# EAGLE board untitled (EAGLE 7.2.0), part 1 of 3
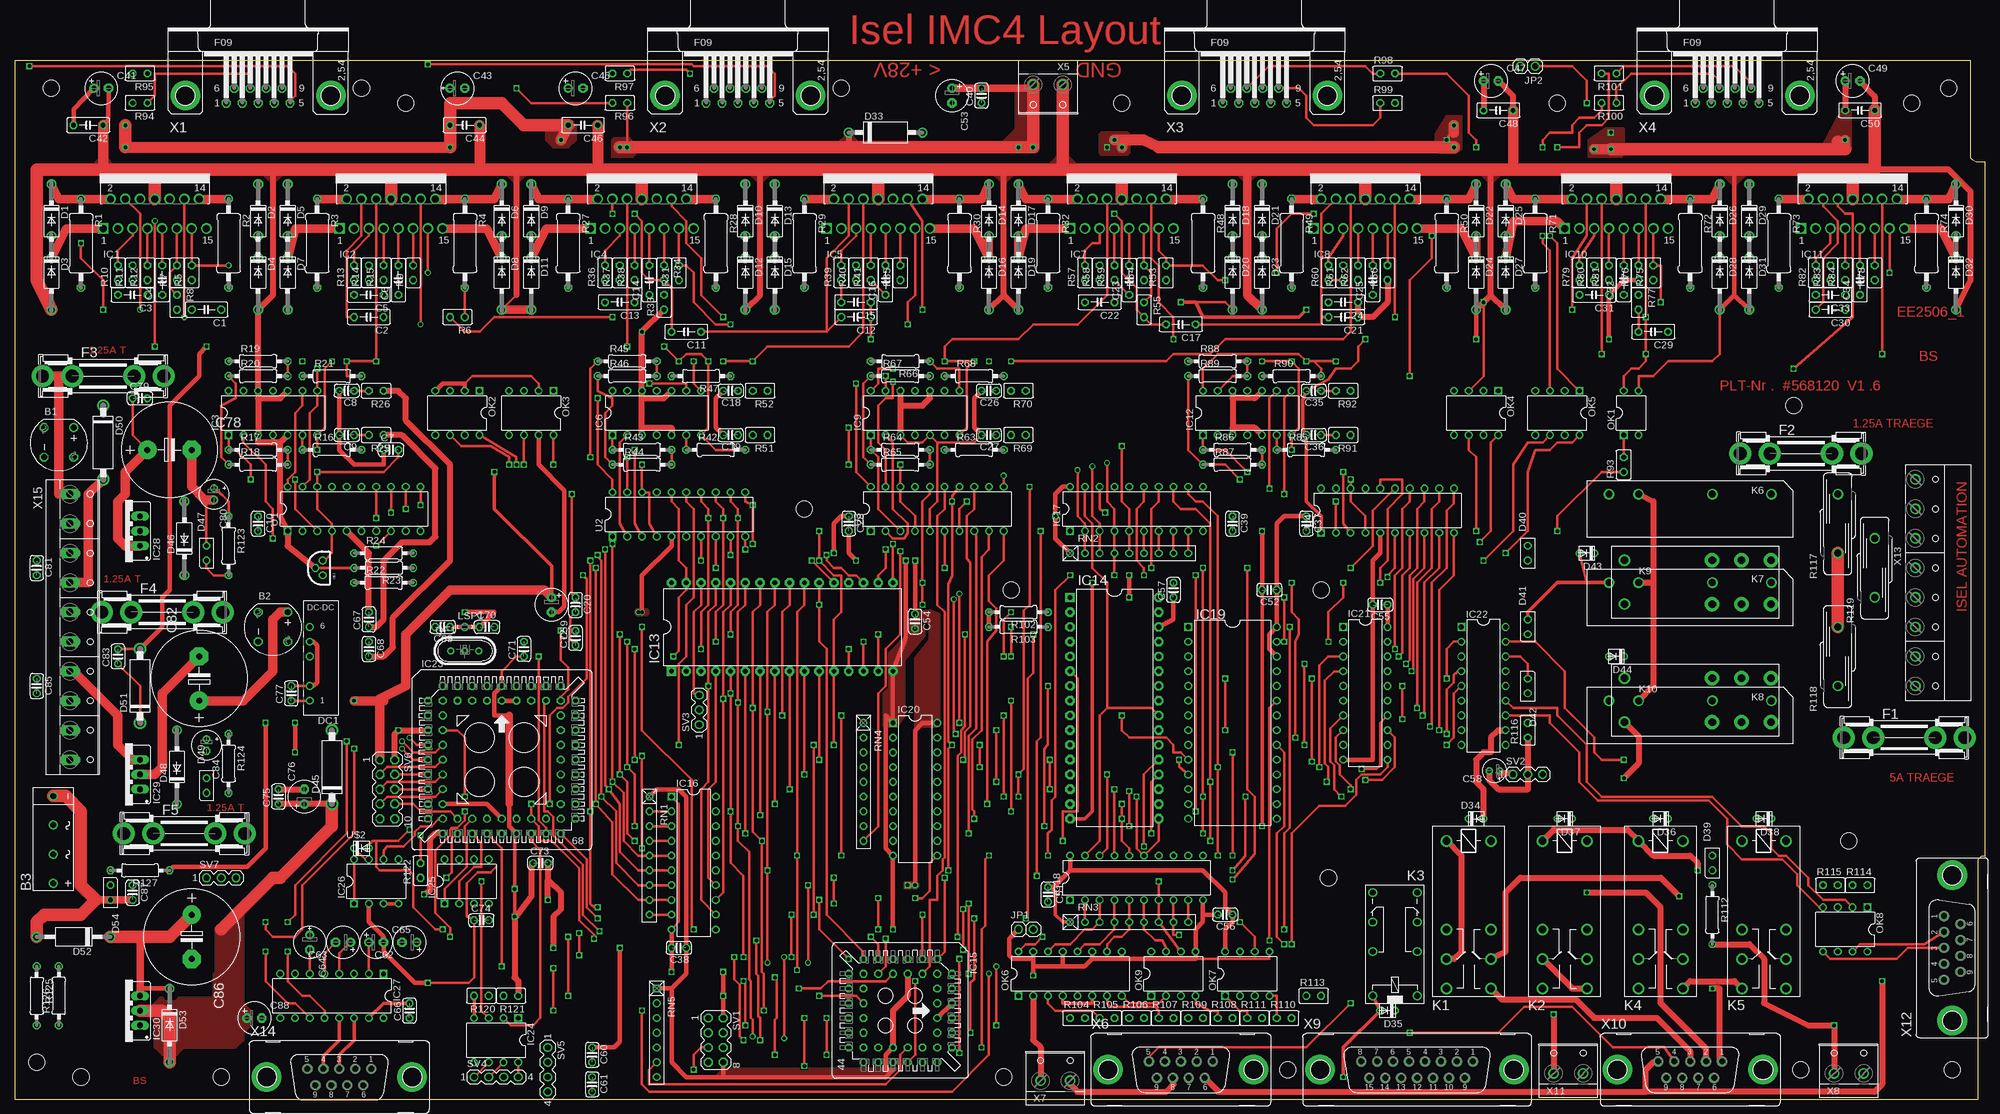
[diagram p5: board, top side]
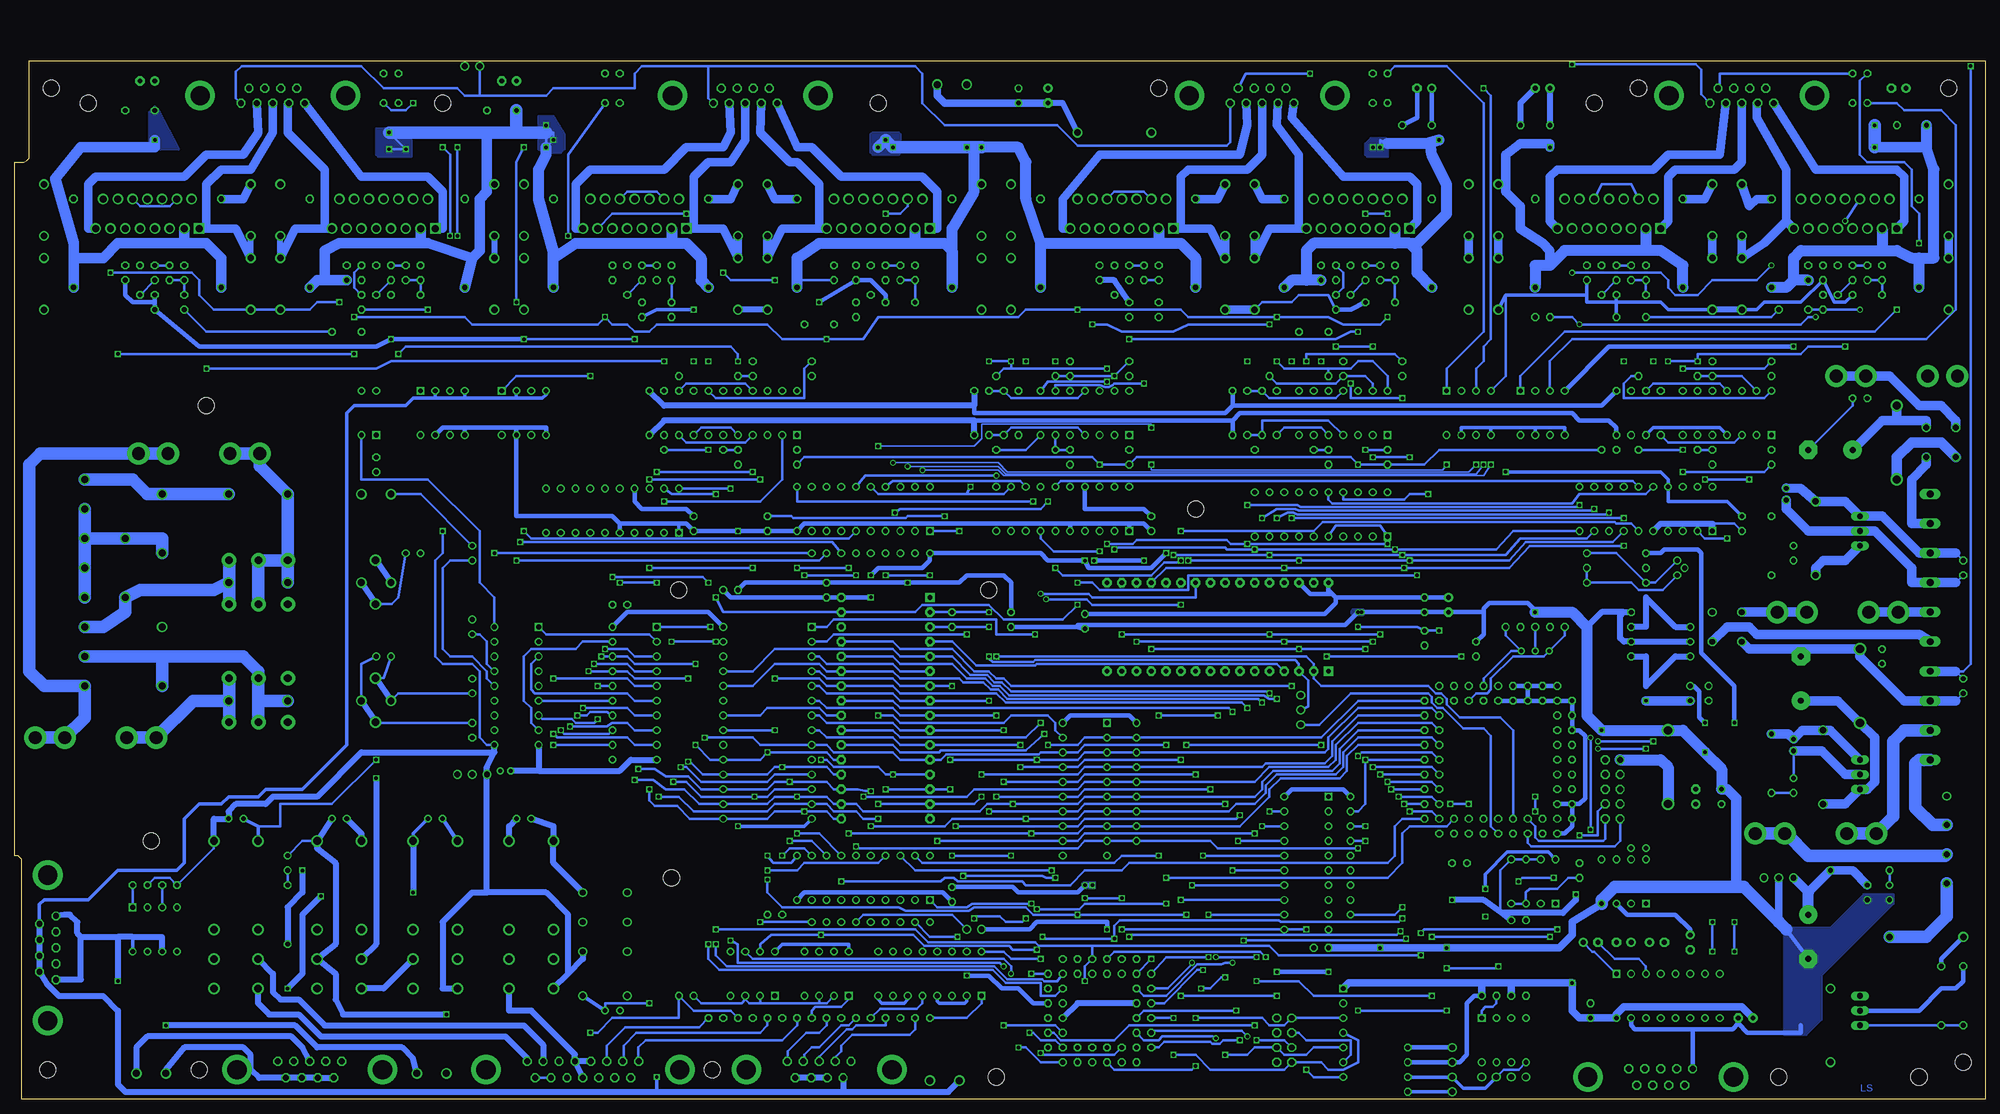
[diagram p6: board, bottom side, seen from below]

Size 339.09 x 178.74 mm. Coordinates in mm from the lower left corner, seen from the top.
Outline: 0,0 337.82,0 337.82,41.28 338.46,41.91 339.09,41.91 339.09,161.29 337.5,161.29 336.87,161.61 336.55,161.93 336.53,162.26 336.53,178.74 0,178.74 0,0
Copper layers (1*16): Top 0.035mm / dielectric 1.5mm / Bottom 0.035mm
Design rules "default": minimum track width 10mil, minimum drill 24mil, track to track 8mil, track to pad 8mil, pad to pad 8mil, via to via 8mil, smd to smd 8mil, copper to edge 40mil, drill to drill 8mil, minimum pad ring 10mil, minimum via ring 8mil, stop-mask expansion 4mil, vias tented up to drill 0mil, thermal gap 10mil
Holes 2.8 mm at 171.45,87.63 224.79,87.63 219.07,5.08 170.18,3.81 307.34,5.08 333.38,5.08 226.06,38.1 35.56,3.81 306.07,119.38 315.6,44.45 326.39,171.45 332.74,173.99 265.43,171.45 142.24,173.99 190.5,171.45 59.69,173.99 67.31,171.45 6.35,173.99 135.89,101.6 3.81,6.35 11.43,3.81

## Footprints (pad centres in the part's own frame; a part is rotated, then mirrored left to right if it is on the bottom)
RB1A = drill 1.016: + -2.54,2.54 | drill 1.016 octagon: - 2.54,-2.54; AC1 2.54,2.54; AC2 -2.54,-2.54
2KBB-R = drill 1.016: + -7.62,0; - 7.391,0; AC1 -2.616,0; AC2 2.413,0
C050-025X075 = drill 0.813 octagon: 1 -2.54,0; 2 2.54,0
C025-024X044 = drill 0.813 octagon: 1 -1.27,0; 2 1.27,0
E2,5-6 = drill 0.813 pad 1.6: + -1.27,0 | drill 0.813 pad 1.6 octagon: - 1.27,0
E2,5-6E = drill 0.813 pad 1.575: + -1.27,0 | drill 0.813 pad 1.575 octagon: - 1.27,0
E1,8-4 = drill 0.711 pad 1.168: + -0.889,0 | drill 0.711 pad 1.168 octagon: - 0.889,0
E7,5-16 = drill 1.016 pad 3.15: + -3.81,0 | drill 1.016 pad 3.15 octagon: - 3.81,0
E2-5 = drill 0.813 pad 1.27: + -1.016,0 | drill 0.813 pad 1.27 octagon: - 1.016,0
DO41-10 = drill 1.118: A 6.35,0; C -6.35,0
DO15-12 = drill 1.118: A 6.35,0; C -6.35,0
DO41-10' = drill 0.8: A 1.27,0; C -1.27,0
U57X32 = drill 0.813: A 1.27,0; K -1.27,0
C1702-15 = drill 1.397: A 5.08,0; C -7.62,0
P1-12E = drill 1.118: A 6.35,0; C -6.35,0
NMA = drill 0.813: 1 0,6.35; 2 0,3.81; 4 0,-1.27; 5 0,-3.81; 6 0,-6.35
SHK20L = drill 2.2 pad 3.81: 1A -10.414,0; 1B -5.334,0; 2A 10.414,0; 2B 5.334,0
MULTIWATT-15 = drill 1.2 square: 1 -8.89,-7.62 | drill 1.2: 2 -7.62,-2.54; 3 -6.35,-7.62; 4 -5.08,-2.54; 5 -3.81,-7.62; 6 -2.54,-2.54; 7 -1.27,-7.62; 8 0,-2.54; 9 1.27,-7.62; 10 2.54,-2.54; 11 3.81,-7.62; 12 5.08,-2.54; 13 6.35,-7.62; 14 7.62,-2.54; 15 8.89,-7.62
DIL14 = drill 0.813 square: 1 -7.62,-3.81 | drill 0.813: 2 -5.08,-3.81; 3 -2.54,-3.81; 4 0,-3.81; 5 2.54,-3.81; 6 5.08,-3.81; 7 7.62,-3.81; 8 7.62,3.81; 9 5.08,3.81; 10 2.54,3.81; 11 0,3.81; 12 -2.54,3.81; 13 -5.08,3.81; 14 -7.62,3.81
DIL32-3 = drill 0.813 pad 1.6 square: 1 -16.51,-7.62 | drill 0.813 pad 1.6 octagon: 2 -13.97,-7.62; 3 -11.43,-7.62; 4 -8.89,-7.62; 5 -6.35,-7.62; 6 -3.81,-7.62; 7 -1.27,-7.62; 8 1.27,-7.62; 9 3.81,-7.62; 10 6.35,-7.62; 11 8.89,-7.62; 12 11.43,-7.62; 13 13.97,-7.62; 14 16.51,-7.62; 15 19.05,-7.62; 16 21.59,-7.62; 17 21.59,7.62; 18 19.05,7.62; 19 16.51,7.62; 20 13.97,7.62; 21 11.43,7.62; 22 8.89,7.62; 23 6.35,7.62; 24 3.81,7.62; 25 1.27,7.62; 26 -1.27,7.62; 27 -3.81,7.62; 28 -6.35,7.62; 29 -8.89,7.62; 30 -11.43,7.62; 31 -13.97,7.62; 32 -16.51,7.62
S44 = drill 0.813: 1 1.27,6.35 | drill 0.813 octagon: 2 -1.27,8.89; 3 -1.27,6.35; 4 -3.81,8.89; 5 -3.81,6.35; 6 -6.35,8.89; 7 -8.89,6.35; 8 -6.35,6.35; 9 -8.89,3.81; 10 -6.35,3.81; 11 -8.89,1.27; 12 -6.35,1.27; 13 -8.89,-1.27; 14 -6.35,-1.27; 15 -8.89,-3.81; 16 -6.35,-3.81; 17 -8.89,-6.35; 18 -6.35,-8.89; 19 -6.35,-6.35; 20 -3.81,-8.89; 21 -3.81,-6.35; 22 -1.27,-8.89; 23 -1.27,-6.35; 24 1.27,-8.89; 25 1.27,-6.35; 26 3.81,-8.89; 27 3.81,-6.35; 28 6.35,-8.89; 29 8.89,-6.35; 30 6.35,-6.35; 31 8.89,-3.81; 32 6.35,-3.81; 33 8.89,-1.27; 34 6.35,-1.27; 35 8.89,1.27; 36 6.35,1.27; 37 8.89,3.81; 38 6.35,3.81; 39 8.89,6.35; 40 6.35,8.89; 41 6.35,6.35; 42 3.81,8.89; 43 3.81,6.35; 44 1.27,8.89
DIL20 = drill 0.813 square: 1 -11.43,-3.81 | drill 0.813: 2 -8.89,-3.81; 3 -6.35,-3.81; 4 -3.81,-3.81; 5 -1.27,-3.81; 6 1.27,-3.81; 7 3.81,-3.81; 8 6.35,-3.81; 9 8.89,-3.81; 10 11.43,-3.81; 11 11.43,3.81; 12 8.89,3.81; 13 6.35,3.81; 14 3.81,3.81; 15 1.27,3.81; 16 -1.27,3.81; 17 -3.81,3.81; 18 -6.35,3.81; 19 -8.89,3.81; 20 -11.43,3.81
DIL28-6 = drill 0.813 square: 1 -16.51,-7.62 | drill 0.813: 2 -13.97,-7.62; 3 -11.43,-7.62; 4 -8.89,-7.62; 5 -6.35,-7.62; 6 -3.81,-7.62; 7 -1.27,-7.62; 8 1.27,-7.62; 9 3.81,-7.62; 10 6.35,-7.62; 11 8.89,-7.62; 12 11.43,-7.62; 13 13.97,-7.62; 14 16.51,-7.62; 15 16.51,7.62; 16 13.97,7.62; 17 11.43,7.62; 18 8.89,7.62; 19 6.35,7.62; 20 3.81,7.62; 21 1.27,7.62; 22 -1.27,7.62; 23 -3.81,7.62; 24 -6.35,7.62; 25 -8.89,7.62; 26 -11.43,7.62; 27 -13.97,7.62; 28 -16.51,7.62
DIL18 = drill 0.813 square: 1 -10.16,-3.81 | drill 0.813: 2 -7.62,-3.81; 3 -5.08,-3.81; 4 -2.54,-3.81; 5 0,-3.81; 6 2.54,-3.81; 7 5.08,-3.81; 8 7.62,-3.81; 9 10.16,-3.81; 10 10.16,3.81; 11 7.62,3.81; 12 5.08,3.81; 13 2.54,3.81; 14 0,3.81; 15 -2.54,3.81; 16 -5.08,3.81; 17 -7.62,3.81; 18 -10.16,3.81
S68 = drill 0.813: 1 0,12.7 | drill 0.813 octagon: 2 0,10.16; 3 -2.54,12.7; 4 -2.54,10.16; 5 -5.08,12.7; 6 -5.08,10.16; 7 -7.62,12.7; 8 -7.62,10.16; 9 -10.16,12.7; 10 -12.7,10.16; 11 -10.16,10.16; 12 -12.7,7.62; 13 -10.16,7.62; 14 -12.7,5.08; 15 -10.16,5.08; 16 -12.7,2.54; 17 -10.16,2.54; 18 -12.7,0; 19 -10.16,0; 20 -12.7,-2.54; 21 -10.16,-2.54; 22 -12.7,-5.08; 23 -10.16,-5.08; 24 -12.7,-7.62; 25 -10.16,-7.62; 26 -12.7,-10.16; 27 -10.16,-12.7; 28 -10.16,-10.16; 29 -7.62,-12.7; 30 -7.62,-10.16; 31 -5.08,-12.7; 32 -5.08,-10.16; 33 -2.54,-12.7; 34 -2.54,-10.16; 35 0,-12.7; 36 0,-10.16; 37 2.54,-12.7; 38 2.54,-10.16; 39 5.08,-12.7; 40 5.08,-10.16; 41 7.62,-12.7; 42 7.62,-10.16; 43 10.16,-12.7; 44 12.7,-10.16; 45 10.16,-10.16; 46 12.7,-7.62; 47 10.16,-7.62; 48 12.7,-5.08; 49 10.16,-5.08; 50 12.7,-2.54; 51 10.16,-2.54; 52 12.7,0; 53 10.16,0; 54 12.7,2.54; 55 10.16,2.54; 56 12.7,5.08; 57 10.16,5.08; 58 12.7,7.62; 59 10.16,7.62; 60 12.7,10.16; 61 10.16,12.7; 62 10.16,10.16; 63 7.62,12.7; 64 7.62,10.16; 65 5.08,12.7; 66 5.08,10.16; 67 2.54,12.7; 68 2.54,10.16
DIL08 = drill 0.813 square: 1 -3.81,-3.81 | drill 0.813: 2 -1.27,-3.81; 3 1.27,-3.81; 4 3.81,-3.81; 5 3.81,3.81; 6 1.27,3.81; 7 -1.27,3.81; 8 -3.81,3.81
DIL16 = drill 0.813 square: 1 -8.89,-3.81 | drill 0.813: 2 -6.35,-3.81; 3 -3.81,-3.81; 4 -1.27,-3.81; 5 1.27,-3.81; 6 3.81,-3.81; 7 6.35,-3.81; 8 8.89,-3.81; 9 8.89,3.81; 10 6.35,3.81; 11 3.81,3.81; 12 1.27,3.81; 13 -1.27,3.81; 14 -3.81,3.81; 15 -6.35,3.81; 16 -8.89,3.81
78XXS = drill 1.016 long: GND 0,-2.54; IN -2.54,-2.54; OUT 2.54,-2.54
317TS = drill 1.016 long: 1 -2.54,-2.54; 2 0,-2.54; 3 2.54,-2.54
1X02 = drill 1.016: 1 -1.27,0; 2 1.27,0
F4052 = drill 1.321: 1 -3.81,3.81; 2 -3.81,-3.81; O1 11.43,-3.81; O2 11.43,3.81; P1 16.51,-3.81; P2 16.51,3.81; S1 21.59,-3.81; S2 21.59,3.81
351 = drill 1.016: 1 -3.81,-3.81; 16 -3.81,3.81; O1 8.89,-3.81; O2 8.89,3.81; P1 3.81,-3.81; P2 3.81,3.81; S1 13.97,-3.81; S2 13.97,3.81
AQ1 = drill 1.2: 1 -15.24,-2.54; 2 -5.08,-2.54; 3 7.62,-2.54; 4 12.7,-2.54
RT2C/O = drill 1.3 pad 2.5: 11 7.56,-3.68; 12 2.52,-3.68; 14 12.6,-3.68; 21 7.56,3.88; 22 2.52,3.88; 24 12.6,3.88 | drill 1.3: A1 -12.6,-3.68; A2 -12.6,3.88
LSP10 = drill 0.813 octagon: MP 0,0
DIL04 = drill 0.813 square: 1 -2.54,-3.81 | drill 0.813: 2 0,-3.81; 3 0,3.81; 4 -2.54,3.81
HC49U = drill 0.7 pad 1.2: 1 -2.413,0; 2 -0.027,0; 3 2.413,0
0411/15 = drill 0.914 octagon: 1 -7.62,0; 2 7.62,0
V526-0 = drill 0.813 octagon: 1 -1.27,0; 2 1.27,0
0207/10 = drill 0.813 octagon: 1 -5.08,0; 2 5.08,0
S20K250 = drill 1.194: 1 0,-5.08; 2 0,5.08
RN-9 = drill 0.813: 1 -10.16,0; 2 -7.62,0; 3 -5.08,0; 4 -2.54,0; 5 0,0; 6 2.54,0; 7 5.08,0; 8 7.62,0; 9 10.16,0
RN-7 = drill 0.813 square: 1 -7.62,0 | drill 0.813: 2 -5.08,0; 3 -2.54,0; 4 0,0; 5 2.54,0; 6 5.08,0; 7 7.62,0
MA04-2 = drill 1.016 octagon: 1 -3.81,-1.27; 2 -3.81,1.27; 3 -1.27,-1.27; 4 -1.27,1.27; 5 1.27,-1.27; 6 1.27,1.27; 7 3.81,-1.27; 8 3.81,1.27
MA03-1 = drill 1.016: 1 -2.54,0; 2 0,0; 3 2.54,0
MA04-1 = drill 1.016: 1 -3.81,0; 2 -1.27,0; 3 1.27,0; 4 3.81,0
MA05-2 = drill 1.016 octagon: 1 -5.08,-1.27; 2 -5.08,1.27; 3 -2.54,-1.27; 4 -2.54,1.27; 5 0,-1.27; 6 0,1.27; 7 2.54,-1.27; 8 2.54,1.27; 9 5.08,-1.27; 10 5.08,1.27
TO-92 = drill 0.813: 1 -1.27,0.318; 2 0,1.587; 3 1.27,0.318
F09HP = drill 1.016 octagon: 1 -5.486,-1.27; 2 -2.743,-1.27; 3 0,-1.27; 4 2.743,-1.27; 5 5.486,-1.27; 6 -4.115,1.27; 7 -1.372,1.27; 8 1.372,1.27; 9 4.115,1.27 | drill 3.302 pad 5.08: G1 -12.522,0; G2 12.522,0
W237-132 = drill 1.194: 1 -2.54,-0.635; 2 2.54,-0.635
F09VP = drill 1.016 octagon: 1 5.486,1.422; 2 2.743,1.422; 3 0,1.422; 4 -2.743,1.422; 5 -5.486,1.422; 6 4.115,-1.422; 7 1.372,-1.422; 8 -1.372,-1.422; 9 -4.115,-1.422 | drill 3.302 pad 5.08: G1 -12.522,0; G2 12.522,0
F15VP = drill 1.016 octagon: 1 9.601,1.422; 2 6.858,1.422; 3 4.115,1.422; 4 1.372,1.422; 5 -1.372,1.422; 6 -4.115,1.422; 7 -6.858,1.422; 8 -9.601,1.422; 9 8.23,-1.422; 10 5.486,-1.422; 11 2.743,-1.422; 12 0,-1.422; 13 -2.743,-1.422; 14 -5.486,-1.422; 15 -8.23,-1.422 | drill 3.302 pad 5.08: G1 -16.662,0; G2 16.662,0
W237-8P = drill 1.194: 1 -17.78,-0.635; 2 -12.7,-0.635; 3 -7.62,-0.635; 4 -2.54,-0.635; 5 2.54,-0.635; 6 7.62,-0.635; 7 12.7,-0.635; 8 17.78,-0.635
W237-10P = drill 1.194 long: 1 -22.86,-0.635; 2 -17.78,-0.635; 3 -12.7,-0.635; 4 -7.62,-0.635; 5 -2.54,-0.635; 6 2.54,-0.635; 7 7.62,-0.635; 8 12.7,-0.635; 9 17.78,-0.635; 10 22.86,-0.635

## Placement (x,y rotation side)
B1  RECTIFIER-RB1A  [RB1A]  7.62,113.03 270 top
B2  RECTIFIER-RB1A  [RB1A]  44.45,81.28 270 top
B3  [2KBB-R]  6.67,44.77 90 top
C1  100n  [C050-025X075]  33.02,135.89 180 top
C2  1n5  [C050-025X075]  60.96,134.62 180 top
C3  100n  [C050-025X075]  20.32,138.43 180 top
C4  47n  [C050-025X075]  25.4,140.97 90 top
C5  100n  [C050-025X075]  60.96,138.43 180 top
C6  47n  [C050-025X075]  66.04,140.97 90 top
C7  [C025-024X044]  64.77,111.76 0 top
C8  [C025-024X044]  57.15,121.92 180 top
C9  [C025-024X044]  57.15,114.3 180 top
C10  [C025-024X044]  41.91,99.06 270 top
C11  100n  [C050-025X075]  115.57,132.08 180 top
C12  1n5  [C050-025X075]  144.78,134.62 180 top
C13  100n  [C050-025X075]  104.14,137.16 180 top
C14  47n  [C050-025X075]  109.22,140.97 90 top
C15  100n  [C050-025X075]  144.78,137.16 180 top
C16  47n  [C050-025X075]  149.86,140.97 90 top
C17  100n  [C050-025X075]  200.66,133.35 180 top
C18  [C025-024X044]  123.19,121.92 180 top
C19  [C025-024X044]  123.19,114.3 180 top
C20  [C025-024X044]  96.52,85.09 270 top
C21  1n5  [C050-025X075]  228.6,134.62 180 top
C22  100n  [C050-025X075]  186.69,137.16 180 top
C23  47n  [C050-025X075]  191.77,140.97 90 top
C24  100n  [C050-025X075]  228.6,137.16 180 top
C25  47n  [C050-025X075]  233.68,140.97 90 top
C26  [C025-024X044]  167.64,121.92 180 top
C27  [C025-024X044]  167.64,114.3 180 top
C28  [C025-024X044]  143.51,99.06 270 top
C29  100n  [C050-025X075]  281.94,132.08 180 top
C30  1n5  [C050-025X075]  312.42,135.89 180 top
C31  100n  [C050-025X075]  271.78,138.43 180 top
C32  47n  [C050-025X075]  276.86,140.97 90 top
C33  100n  [C050-025X075]  312.42,138.43 180 top
C34  47n  [C050-025X075]  317.5,140.97 90 top
C35  [C025-024X044]  223.52,121.92 180 top
C36  [C025-024X044]  223.52,114.3 180 top
C37  [C025-024X044]  222.25,99.06 270 top
C38  [C025-024X044]  114.3,26.04 180 top
C39  [C025-024X044]  209.55,99.06 270 top
C40  [C025-024X044]  166.37,172.72 90 top
C41  [E2,5-6]  14.92,173.99 0 top
C42  [C050-025X075]  12.7,167.64 180 top
C43  [E2,5-6E]  76.2,173.99 0 top
C44  [C050-025X075]  77.47,167.64 180 top
C45  [E2,5-6]  96.52,173.99 0 top
C46  [C050-025X075]  97.79,167.64 180 top
C47  [E2,5-6]  254,175.26 0 top
C48  [C050-025X075]  255.27,170.18 180 top
C49  [E2,5-6]  316.23,175.26 0 top
C50  [C050-025X075]  317.5,170.18 180 top
C51  [C025-024X044]  177.8,35.24 270 top
C52  [C025-024X044]  215.9,87.63 180 top
C53  [E2,5-6]  161.29,172.72 270 top
C54  [C025-024X044]  154.94,82.23 270 top
C55  [C025-024X044]  234.95,85.09 180 top
C56  [C025-024X044]  208.28,31.75 180 top
C57  [C025-024X044]  199.39,87.63 90 top
C58  [E1,8-4]  254.63,56.52 180 top
C59  [E2,5-6]  92.39,85.09 270 top
C60  [C025-024X044]  99.38,7.62 270 top
C61  [C025-024X044]  99.38,2.54 270 top
C62  [E2,5-6]  67.95,26.99 180 top
C63  [E2,5-6]  56.52,26.99 180 top
C64  [E2,5-6E]  50.8,26.99 270 top
C65  [E2,5-6]  62.23,26.99 0 top
C66  [C025-024X044]  67.95,15.24 90 top
C67  [C025-024X044]  60.96,82.55 90 top
C68  [C025-024X044]  60.96,77.47 270 top
C69  22pF  [C025-024X044]  73.66,81.28 180 top
C70  22pF  [C025-024X044]  81.28,81.28 0 top
C71  [C025-024X044]  87.63,77.47 90 top
C72  [C025-024X044]  96.52,79.38 90 top
C73  [C025-024X044]  90.49,40.64 0 top
C74  [C025-024X044]  80.33,30.8 0 top
C75  [C025-024X044]  45.4,52.07 90 top
C76  [E2,5-6]  49.85,52.07 90 top
C77  [C025-024X044]  47.62,69.85 90 top
C78  [E7,5-16]  26.67,111.76 0 top
C79  [C025-024X044]  21.59,120.65 0 top
C80  [E2-5]  34.29,104.14 270 top
C81  [C025-024X044]  3.81,91.44 270 top
C82  [E7,5-16]  31.75,72.39 90 top
C83  [C025-024X044]  17.78,76.2 90 top
C84  [E2-5]  33.02,60.96 270 top
C85  [C025-024X044]  3.81,71.12 270 top
C86  [E7,5-16]  30.48,27.94 270 top
C87  [C025-024X044]  20.32,35.56 270 top
C88  [E2,5-6]  41.27,13.97 0 top
D1  MUR150RL  [DO41-10]  6.35,151.13 270 top
D2  MUR150RL  [DO41-10]  41.91,151.13 270 top
D3  MUR150RL  [DO41-10]  6.35,142.24 270 top
D4  MUR150RL  [DO41-10]  41.91,142.24 270 top
D5  MUR150RL  [DO41-10]  46.99,151.13 270 top
D6  MUR150RL  [DO41-10]  83.82,151.13 270 top
D7  MUR150RL  [DO41-10]  46.99,142.24 270 top
D8  MUR150RL  [DO41-10]  83.82,142.24 270 top
D9  MUR150RL  [DO41-10]  88.9,151.13 270 top
D10  MUR150RL  [DO41-10]  125.73,151.13 270 top
D11  MUR150RL  [DO41-10]  88.9,142.24 270 top
D12  MUR150RL  [DO41-10]  125.73,142.24 270 top
D13  MUR150RL  [DO41-10]  130.81,151.13 270 top
D14  MUR150RL  [DO41-10]  167.64,151.13 270 top
D15  MUR150RL  [DO41-10]  130.81,142.24 270 top
D16  MUR150RL  [DO41-10]  167.64,142.24 270 top
D17  MUR150RL  [DO41-10]  172.72,151.13 270 top
D18  MUR150RL  [DO41-10]  209.55,151.13 270 top
D19  MUR150RL  [DO41-10]  172.72,142.24 270 top
D20  MUR150RL  [DO41-10]  209.55,142.24 270 top
D21  MUR150RL  [DO41-10]  214.63,151.13 270 top
D22  MUR150RL  [DO41-10]  251.46,151.13 270 top
D23  MUR150RL  [DO41-10]  214.63,142.24 270 top
D24  MUR150RL  [DO41-10]  251.46,142.24 270 top
D25  MUR150RL  [DO41-10]  256.54,151.13 270 top
D26  MUR150RL  [DO41-10]  293.37,151.13 270 top
D27  MUR150RL  [DO41-10]  256.54,142.24 270 top
D28  MUR150RL  [DO41-10]  293.37,142.24 270 top
D29  MUR150RL  [DO41-10]  298.45,151.13 270 top
D30  MUR150RL  [DO41-10]  334.01,151.13 270 top
D31  MUR150RL  [DO41-10]  298.45,142.24 270 top
D32  MUR150RL  [DO41-10]  334.01,142.24 270 top
D33  1N5060GP  [DO15-12]  149.86,166.37 0 top
D34  1N4004  [DO41-10']  251.46,48.26 0 top
D35  1N4004  [DO41-10']  236.22,15.24 180 top
D36  1N4004  [DO41-10']  283.21,48.26 180 top
D37  1N4004  [DO41-10']  266.7,48.26 180 top
D38  1N4004  [DO41-10']  300.99,48.26 180 top
D39  U57X32  [U57X32]  292.1,40.64 90 top
D40  U57X32  [U57X32]  260.35,93.98 90 top
D41  U57X32  [U57X32]  260.35,81.28 90 top
D42  U57X32  [U57X32]  260.35,71.12 270 top
D43  1N4004  [DO41-10']  270.51,93.98 180 top
D44  1N4004  [DO41-10']  275.59,76.2 180 top
D45  P6KEXXA  [C1702-15]  54.61,58.42 90 top
D46  1N4004  [DO41-10]  29.21,96.52 90 top
D47  U57X32  [U57X32]  33.02,93.98 90 top
D48  1N4004  [DO41-10]  27.94,57.15 90 top
D49  U57X32  [U57X32]  33.02,53.98 90 top
D50  P6KEXXA  [C1702-15]  15.24,111.76 270 top
D51  P6KEXXA  [C1702-15]  21.59,72.39 90 top
D52  BZW06-28  [P1-12E]  10.16,27.94 180 top
D53  1N4004  [DO41-10]  26.67,12.7 270 top
D54  U57X32  [U57X32]  16.51,35.56 270 top
DC1  [NMA]  50.8,74.93 180 top
F1  [SHK20L]  325.12,62.23 0 top
F2  [SHK20L]  307.34,111.12 0 top
F3  [SHK20L]  15.24,124.46 0 top
F4  [SHK20L]  25.4,83.82 0 top
F5  [SHK20L]  29.21,45.72 0 top
IC1  L292  [MULTIWATT-15]  24.13,157.48 0 top
IC2  L292  [MULTIWATT-15]  64.77,157.48 0 top
IC3  TLE2064P  [DIL14]  44.45,118.11 0 top
IC4  L292  [MULTIWATT-15]  107.95,157.48 0 top
IC5  L292  [MULTIWATT-15]  148.59,157.48 0 top
IC6  TLE2064P  [DIL14]  110.49,118.11 0 top
IC7  L292  [MULTIWATT-15]  190.5,157.48 0 top
IC8  L292  [MULTIWATT-15]  232.41,157.48 0 top
IC9  TLE2064P  [DIL14]  154.94,118.11 0 top
IC10  L292  [MULTIWATT-15]  275.59,157.48 0 top
IC11  L292  [MULTIWATT-15]  316.23,157.48 0 top
IC12  TLE2064P  [DIL14]  212.09,118.11 0 top
IC13  AM29F010P  [DIL32-3]  129.54,81.28 0 top
IC14  AM29F010P  [DIL32-3]  189.23,69.85 270 top
IC15  [S44]  152.4,15.24 270 top
IC16  74HCT573N  [DIL20]  116.84,40.64 270 top
IC17  74HCT540N  [DIL20]  193.04,101.6 0 top
IC18  74HCT540N  [DIL20]  193.04,38.1 0 top
IC19  [DIL28-6]  209.55,64.77 270 top
IC20  74HCT573N  [DIL20]  154.94,53.34 270 top
IC21  74273N  [DIL20]  232.41,69.85 270 top
IC22  [DIL18]  252.73,71.12 270 top
IC23  [S68]  83.82,58.42 0 top
IC24  [DIL08]  82.87,10.16 180 top
IC25  [DIL08]  77.79,37.47 0 top
IC26  MAX705CPA  [DIL08]  62.23,37.47 0 top
IC27  MAX232  [DIL16]  54.61,17.78 180 top
IC28  [78XXS]  19.05,97.79 90 top
IC29  [78XXS]  19.05,55.88 90 top
IC30  [317TS]  19.05,15.24 90 top
JP1  [1X02]  173.99,29.21 0 top
JP2  [1X02]  260.35,177.8 180 top
K1  4052  [F4052]  250.19,40.64 270 top
K2  4052  [F4052]  266.7,40.64 270 top
K3  351  [351]  237.49,21.59 90 top
K4  4052  [F4052]  283.21,40.64 270 top
K5  4052  [F4052]  300.99,40.64 270 top
K6  AQ2A2-ZP3  [AQ1]  287.02,101.6 180 top
K7  AQ2A2-ZP3  [AQ1]  287.02,86.36 180 top
K8  AQ2A2-ZP3  [AQ1]  287.02,66.04 180 top
K9  RT424A12  [RT2C/O]  289.56,88.9 0 top
K10  RT424A12  [RT2C/O]  289.56,68.58 0 top
LSP1  LSP10  [LSP10]  77.47,81.28 0 top
OK1  TLP523  [DIL04]  279.4,118.11 0 top
OK2  ILD621  [DIL08]  76.2,118.11 180 top
OK3  ILD621  [DIL08]  88.9,118.11 180 top
OK4  ILD621  [DIL08]  251.46,118.11 180 top
OK5  ILD621  [DIL08]  265.43,118.11 180 top
OK6  TLP621-4DIL16  [DIL16]  181.61,21.59 0 top
OK7  HCPL2530  [DIL08]  212.09,21.59 0 top
OK8  ILD621  [DIL08]  314.96,29.21 180 top
OK9  HCPL2530  [DIL08]  199.39,21.59 0 top
QF1  8M10AHC49T  [HC49U]  77.47,77.15 0 top
R1  2R2  [0411/15]  11.43,147.32 270 top
R2  2R2  [0411/15]  36.83,147.32 270 top
R3  2R2  [0411/15]  52.07,147.32 270 top
R4  2R2  [0411/15]  77.47,147.32 270 top
R5  15K  [V526-0]  30.48,142.24 90 top
R6  15K  [V526-0]  76.2,134.62 180 top
R7  15K  [V526-0]  27.94,142.24 90 top
R8  100K  [V526-0]  27.94,137.16 270 top
R9  15K  [V526-0]  68.58,142.24 90 top
R10  510R  [V526-0]  17.78,142.24 90 top
R11  510R  [V526-0]  20.32,142.24 90 top
R12  22K  [V526-0]  22.86,142.24 90 top
R13  510R  [V526-0]  58.42,142.24 90 top
R14  510R  [V526-0]  60.96,142.24 90 top
R15  22K  [V526-0]  63.5,142.24 90 top
R16  20K  [0207/10]  54.61,111.76 0 top
R17  4K99 50ppm/K  [0207/10]  41.91,111.76 0 top
R18  10K  [0207/10]  41.91,109.22 0 top
R19  4K99 50ppm/K  [0207/10]  41.91,127 0 top
R20  10K  [0207/10]  41.91,124.46 0 top
R21  20K  [0207/10]  54.61,124.46 0 top
R22  6K19  [0207/10]  63.5,88.9 0 top
R23  7K5  [0207/10]  63.5,91.44 180 top
R24  270R  [0207/10]  63.5,93.98 0 top
R25  10R  [V526-0]  62.23,114.3 180 top
R26  10R  [V526-0]  62.23,121.92 180 top
R27  2R2  [0411/15]  95.25,147.32 270 top
R28  2R2  [0411/15]  120.65,147.32 270 top
R29  2R2  [0411/15]  135.89,147.32 270 top
R30  2R2  [0411/15]  162.56,147.32 270 top
R31  15K  [V526-0]  114.3,142.24 90 top
R32  2R2  [0411/15]  177.8,147.32 270 top
R33  15K  [V526-0]  111.76,137.16 90 top
R34  100K  [V526-0]  111.76,142.24 270 top
R35  15K  [V526-0]  152.4,142.24 90 top
R36  510R  [V526-0]  101.6,142.24 90 top
R37  510R  [V526-0]  104.14,142.24 90 top
R38  22K  [V526-0]  106.68,142.24 90 top
R39  510R  [V526-0]  142.24,142.24 90 top
R40  510R  [V526-0]  144.78,142.24 90 top
R41  22K  [V526-0]  147.32,142.24 90 top
R42  20K  [0207/10]  120.65,111.76 0 top
R43  4K99 50ppm/K  [0207/10]  107.95,111.76 0 top
R44  10K  [0207/10]  107.95,109.22 0 top
R45  4K99 50ppm/K  [0207/10]  105.41,127 0 top
R46  10K  [0207/10]  105.41,124.46 0 top
R47  20K  [0207/10]  118.11,124.46 180 top
R48  2R2  [0411/15]  204.47,147.32 270 top
R49  2R2  [0411/15]  219.71,147.32 270 top
R50  2R2  [0411/15]  246.38,147.32 270 top
R51  10R  [V526-0]  128.27,114.3 180 top
R52  10R  [V526-0]  128.27,121.92 180 top
R53  15K  [V526-0]  198.12,142.24 90 top
R54  15K  [V526-0]  194.31,142.24 90 top
R55  100K  [V526-0]  194.31,135.89 270 top
R56  15K  [V526-0]  236.22,142.24 90 top
R57  510R  [V526-0]  184.15,142.24 90 top
R58  510R  [V526-0]  186.69,142.24 90 top
R59  22K  [V526-0]  189.23,142.24 90 top
R60  510R  [V526-0]  226.06,142.24 90 top
R61  510R  [V526-0]  228.6,142.24 90 top
R62  22K  [V526-0]  231.14,142.24 90 top
R63  20K  [0207/10]  165.1,111.76 0 top
R64  4K99 50ppm/K  [0207/10]  152.4,111.76 0 top
R65  10K  [0207/10]  152.4,109.22 0 top
R66  4K99 50ppm/K  [0207/10]  152.4,127 180 top
R67  10K  [0207/10]  152.4,124.46 0 top
R68  20K  [0207/10]  165.1,124.46 0 top
R69  10R  [V526-0]  172.72,114.3 180 top
R70  10R  [V526-0]  172.72,121.92 180 top
R71  2R2  [0411/15]  261.62,147.32 270 top
R72  2R2  [0411/15]  288.29,147.32 270 top
R73  2R2  [0411/15]  303.53,147.32 270 top
R74  2R2  [0411/15]  328.93,147.32 270 top
R75  15K  [V526-0]  281.94,142.24 90 top
R76  15K  [V526-0]  279.4,142.24 90 top
R77  100K  [V526-0]  279.4,137.16 270 top
R78  15K  [V526-0]  320.04,142.24 90 top
R79  510R  [V526-0]  269.24,142.24 90 top
R80  510R  [V526-0]  271.78,142.24 90 top
R81  22K  [V526-0]  274.32,142.24 90 top
R82  510R  [V526-0]  309.88,142.24 90 top
R83  510R  [V526-0]  312.42,142.24 90 top
R84  22K  [V526-0]  314.96,142.24 90 top
R85  20K  [0207/10]  222.25,111.76 0 top
R86  4K99 50ppm/K  [0207/10]  209.55,111.76 0 top
R87  10K  [0207/10]  209.55,109.22 0 top
R88  4K99 50ppm/K  [0207/10]  207.01,127 0 top
R89  10K  [0207/10]  207.01,124.46 0 top
R90  20K  [0207/10]  219.71,124.46 0 top
R91  10R  [V526-0]  228.6,114.3 180 top
R92  10R  [V526-0]  228.6,121.92 180 top
R93  1K  [V526-0]  276.86,109.22 90 top
R94  2K2  [V526-0]  21.59,171.45 180 top
R95  2K2  [V526-0]  21.59,176.53 180 top
R96  2K2  [V526-0]  104.14,171.45 180 top
R97  2K2  [V526-0]  104.14,176.53 180 top
R98  2K2  [V526-0]  236.22,176.53 0 top
R99  2K2  [V526-0]  236.22,171.45 0 top
R100  2K2  [V526-0]  274.32,171.45 180 top
R101  2K2  [V526-0]  274.32,176.53 180 top
R102  10K  [0207/10]  172.72,83.82 180 top
R103  10K  [0207/10]  172.72,81.28 180 top
R104  2K2  [V526-0]  182.88,13.97 0 top
R105  2K2  [V526-0]  187.96,13.97 0 top
R106  2K2  [V526-0]  193.04,13.97 0 top
R107  2K2  [V526-0]  198.12,13.97 0 top
R108  1K6  [V526-0]  208.28,13.97 0 top
R109  1K6  [V526-0]  203.2,13.97 0 top
R110  1K6  [V526-0]  218.44,13.97 0 top
R111  1K6  [V526-0]  213.36,13.97 0 top
R112  4K7  [0207/10]  292.1,31.75 270 top
R113  2K2  [V526-0]  223.52,17.78 0 top
R114  1K  [V526-0]  317.5,36.83 0 top
R115  1K  [V526-0]  312.42,36.83 0 top
R116  NC  [V526-0]  260.35,63.5 90 top
R117  S20K250  [S20K250]  313.69,99.06 0 top
R118  S20K250  [S20K250]  313.69,76.2 0 top
R119  S20K250  [S20K250]  320.04,91.44 0 top
R120  2K2  [V526-0]  80.33,17.78 180 top
R121  2K2  [V526-0]  85.41,17.78 180 top
R122  1K  [V526-0]  69.85,39.37 90 top
R123  [0207/10]  36.83,95.25 270 top
R124  [0207/10]  36.83,57.79 270 top
R125  249R  [0207/10]  3.81,17.78 270 top
R126  750R  [0207/10]  7.62,17.78 90 top
R127  [0207/10]  21.59,39.37 180 top
RN1  47K  [RN-9]  109.22,41.91 270 top
RN2  47K  [RN-9]  191.77,93.98 0 top
RN3  47K  [RN-9]  191.77,30.48 0 top
RN4  47K  [RN-9]  146.05,54.61 270 top
RN5  [RN-7]  110.49,11.43 270 top
SV1  [MA04-2]  120.65,10.16 270 top
SV2  [MA03-1]  260.35,55.88 0 top
SV3  [MA03-1]  117.79,66.99 90 top
SV4  [MA04-1]  82.87,3.81 0 top
SV5  [MA04-1]  91.76,5.08 270 top
SV6  [MA05-2]  64.14,53.34 270 top
SV7  [MA03-1]  35.56,38.1 0 top
U1  TLC7528DIL20  [DIL20]  58.42,101.6 0 top
U2  TLC7528DIL20  [DIL20]  114.3,100.65 0 top
U3  TLC7528DIL20  [DIL20]  158.75,101.6 0 top
U4  TLC7528DIL20  [DIL20]  236.22,101.28 0 top
U$1  TL431  [TO-92]  53.34,91.44 90 top
U$2  SB030  [DO41-10']  59.69,43.18 0 top
X1  [F09HP]  41.91,172.72 0 top
X2  [F09HP]  124.46,172.72 0 top
X3  [F09HP]  213.36,172.72 0 top
X4  [F09HP]  294.64,172.72 0 top
X5  [W237-132]  177.8,173.99 180 top
X6  [F09VP]  200.66,5.08 0 top
X7  [W237-132]  179.07,3.81 0 top
X8  [W237-132]  315.6,5.08 0 top
X9  [F15VP]  241.3,5.08 0 top
X10  [F09VP]  288.29,5.08 0 top
X11  [W237-132]  267.34,5.08 0 top
X12  [F09VP]  333.38,26.04 90 top
X13  [W237-8P]  327.66,88.9 270 top
X14  [F09VP]  55.88,3.81 0 top
X15  [W237-10P]  10.16,81.28 270 top

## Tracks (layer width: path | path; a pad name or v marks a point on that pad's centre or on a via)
+5V  (via drill 0.6)
  Top 0.406: SV3.3 117.16,69.53 116.84,69.85 116.84,83.82 118.11,85.09 IC13.30 | 85.09,66.04 85.09,46.99 | v95.89,104.14 95.89,87 C20.1 | C71.1 86.36,76.2 83.82,73.66 IC23.1 | v71.12,20 78.11,20 79.06,20.96 C74.1 77.79,31.43 77.79,37.15 79.69,39.05 81.92,39.05 82.87,40.01 | C77.1 DC1.1
  Top 0.61: v82.55,107.95 82.55,101.6 92.39,91.76 C59.+ | RN3.1 180.34,30.48 179.07,31.75 179.07,35.88 C51.1 | 86.04,46.04 v86.04,36.2 v86.04,31.43
  Top 0.813: C37.1 218.44,100.33 217.17,99.06 C52.1 IC19.28 215.9,80.01 215.9,77.47 IC19.26 | C28.1 142.24,100.33 140.97,99.06 v140.97,93.98 | C54.1 v154.94,92.71 | RN2.1 179.07,96.52 v179.07,100.33 179.07,104.14 180.34,105.41 IC17.20 | C55.1 IC21.20 | IC14.30 199.39,82.55 C57.1 | v191.77,86.36 v191.77,90.17 | IC18.20 181.61,39.37 | 181.61,39.37 178.75,36.51 C51.1 | v153.67,36.83 v154.94,36.83 154.94,63.5 156.21,64.77 IC20.20 | 113.03,19.05 115.57,21.59 C38.1 115.57,52.07 114.3,53.34 110.49,53.34 RN1.1 | 121.92,3.81 115.57,3.81 113.03,6.35 113.03,19.05 | SV1.8 121.92,3.81 | 121.92,3.81 149.86,3.81 151.13,5.08 149.86,5.08 149.86,7.62 IC15.34 | 181.61,39.37 204.47,39.37 208.28,35.56 208.28,33.02 C56.1 209.55,30.48 208.28,29.21 OK7.8 | 85.09,50.8 85.09,46.99 86.04,46.04 IC23.37 | IC23.1 82.55,69.85 82.55,66.04 85.09,66.04 | 113.03,19.05 RN5.1 | IC26.2 60.96,30.48 63.5,27.94 C65.- 63.5,25.4 68.9,20 v71.12,20
  Top 1.016: IC15.12 153.67,17.78 151.13,15.24 IC15.34 | v86.04,31.43 86.04,31.12 | 86.04,31.12 86.04,20.96 86.68,20.32 R121.1 | C73.1 88.9,40.32 88.9,34.93 86.04,31.12 | D45.C C76.+ C75.1
  Top 1.27: 85.09,66.04 85.09,50.8
  Top 1.676: SV6.1 62.86,68.9 | 62.86,68.9 63.5,68.58 v58.42,68.58 | 62.86,68.9 67.31,71.12 67.31,80.01 74.93,87.63 91.12,87.63 C59.+
  Top 2.184: IC30.2 25.4,15.24 26.67,13.97 D53.A | D45.C 54.61,46.99 45.72,38.1 44.45,38.1 35.56,29.21
  Bottom 0.406: U2.17 110.49,103.19 100.01,103.19 99.06,104.14 v95.89,104.14 | C39.1 205.42,100.33 205.1,100.01 185.74,100.01 185.42,100.33 v179.07,100.33 | 84.14,20 86.68,20.32
  Bottom 0.61: C10.1 44.45,102.87 54.61,102.87 U1.17 54.61,106.68 55.88,107.95 v82.55,107.95 | OK7.8 207.01,26.67 195.58,26.67 OK9.8 | IC25.8 75.25,42.55 82.23,42.55 86.04,38.74 v86.04,36.2
  Bottom 0.813: U3.17 154.94,101.6 144.78,101.6 C28.1 | C37.1 223.52,101.6 231.14,101.6 232.41,102.87 U4.17 | v140.97,93.98 143.51,91.44 154.3,91.44 v154.94,92.71 161.29,92.71 162.56,93.98 RN2.1 181.61,92.71 182.88,91.44 190.5,91.44 v191.77,90.17 | RN4.1 147.32,66.04 157.48,66.04 IC20.20 | IC16.20 119.38,53.34 110.49,53.34 RN1.1 | IC21.20 233.68,83.82 219.71,83.82 IC19.28 | C52.1 215.9,86.36 C57.1 IC14.32 v191.77,86.36 | IC13.32 113.03,87.63 | 113.03,87.63 112.39,87 | 111.76,86.36 C20.1 C59.+ | IC13.30 116.2,87 113.03,87 | 113.03,87.63 113.03,87 | 113.03,87 112.39,87 | 112.39,87 111.76,86.36 | 111.76,86.36 111.76,85.41 113.67,83.5 C54.1 | v153.67,36.83 v154.94,36.83 156.21,35.56 166.37,35.56 167.32,36.51 C51.1 | C60.2 SV5.2 90.49,6.35 89.22,7.62 89.22,16.51 87.95,17.78 R121.1 | R125.1 3.81,20.32 5.08,19.05 7.62,19.05 11.43,15.24 IC30.2
  Bottom 1.27: RN5.1 109.54,20 86.68,20 | R121.1 86.68,20 | 86.68,20 84.14,20 81.6,20 | R120.1 81.6,20 | 81.6,20 v71.12,20 71.12,15.24 69.85,13.97 C66.1 IC27.16 63.5,14.61 62.23,15.88 41.91,15.88 C88.+
  Bottom 1.676: DC1.1 v58.42,68.58
  Bottom 1.93: SV6.1 55.88,58.42 54.61,57.15 D45.C
  other vias: 143.51,100.33 217.17,87.63 110.49,19.05
  pour Top (no thermals): 155.26,83.82 155.26,83.19 157.48,81.92 157.48,79.06 154.94,75.88 154.94,63.82 155.57,63.82 155.89,64.14 158.75,64.14 159.07,64.45 159.07,83.5 157.48,84.14
  pour Top: 153.03,37.47 153.03,36.2 155.26,36.2 155.57,36.51 155.57,37.15 155.26,37.47
  pour Bottom: 153.03,37.47 153.03,36.2 155.26,36.2 155.57,36.51 155.57,37.15 155.26,37.47
  pour Top: 121.92,5.4 120.02,3.49 150.18,3.49 151.76,5.08 151.76,5.4
  pour Top (no thermals): 22.86,15.24 25.08,17.46 25.4,17.46 25.72,16.83 27.62,16.83 28.26,17.46 34.29,17.46 34.29,21.59 34.61,21.91 34.61,29.53 39.37,34.29 39.37,16.51 40.64,15.24 40.64,12.7 39.37,11.43 39.37,10.16 38.1,8.89 29.21,8.89 27.94,7.62 25.4,7.62 24.13,8.89 24.13,13.34 22.86,14.61
+12V
  Top 1.016: C67.1 62.23,81.28 63.5,82.55 63.5,92.71 66.67,95.89 71.44,95.89 72.39,96.84 72.39,108.59 66.67,114.3 R25.1
  Bottom 0.813: R25.1 63.5,115.57 64.77,116.84 69.85,116.84 71.12,118.11 128.27,118.11 129.54,116.84 | 129.54,116.84 R51.1 | 129.54,116.84 173.99,116.84
  Bottom 1.016: R69.1 173.99,116.84 227.33,116.84 R91.1 | DC1.6 53.34,81.28 58.42,86.36 58.42,81.28 C67.1
+24V  (via drill 0.6)
  Top 0.406: X2.5 129.95,171.86 130.81,172.72 130.81,176.53 129.54,177.8 116.84,177.8 116.52,178.12 v71.12,178.12 | X1.5 47.4,171.86 48.26,172.72 48.26,176.53 46.99,177.8 v2.54,177.8
  Top 1.676: IC29.OUT 20.32,58.42 17.78,60.96 17.78,66.04 10.16,73.66 X15.7
  Bottom 0.406: X4.5 300.99,172.31 300.99,176.85 300.04,177.8 279.4,177.8 275.59,173.99 262.89,173.99 261.62,172.72 259.08,172.72 | 259.08,172.72 247.65,172.72 246.38,173.99 232.41,173.99 232.41,176.53 231.14,177.8 219.71,177.8 | 219.71,177.8 184.15,177.8 182.88,176.53 182.88,171.45 179.07,167.64 159.7,167.64 156.21,164.15 130.49,164.15 129.95,164.69 X2.5 | X3.5 219.71,172.31 219.71,177.8 | JP2.2 259.08,172.72 | v71.12,178.12 49.85,178.12 48.9,177.17 48.9,172.95 X1.5 | C85.1 5.08,73.66 3.81,73.66 2.54,74.93 v2.54,177.8
  Bottom 1.676: IC29.OUT 26.67,63.5 D48.A 31.5,63.5 C84.+ 33.91,62.87 R124.1 | X15.7 5.08,73.66
+UB  (via drill 0.6)
  Top 0.406: R6.1 R4.2 | R96.1 v105.41,163.83 | v246.38,165.1 v247.65,167.64
  Top 0.813: C41.+ 10.16,170.43 C42.2 | C44.2 74.93,171.45
  Top 1.016: D33.C 143.51,163.83 | C47.+ C48.2 | C49.+ C50.2
  Top 1.27: C53.+ C40.2 175.26,173.99 X5.2
  Top 1.778: v274.64,163.51 v271.78,163.51 | 247.65,166.37 v247.65,167.64 | 314.96,163.51 v314.96,165.1
  Top 1.93: v19.05,163.83 v74.93,163.83 C44.2 | C46.2 v93.98,165.1 | 190.5,165.1 194.31,165.1 196.85,163.83 | 190.5,165.1 190.5,163.83 | 190.5,165.1 v189.23,165.1
  Top 2.184: v19.05,167.64 v19.05,163.83 | v74.93,163.83 74.93,171.45 83.82,171.45 87.63,167.64 C46.2 | v104.14,163.83 v105.41,163.83 143.51,163.83 v172.72,163.83 v175.26,163.83 X5.2 | v247.65,163.83 196.85,163.83 | v274.64,163.51 314.96,163.51 313.69,164.78
  Bottom 0.406: R48.2 204.47,140.97 R53.1 | 15.24,146.05 13.97,146.05 12.7,144.78 | 102.87,164.47 104.14,165.1 v104.14,163.83 | R50.2 246.38,146.05 | 248.92,160.02 v247.65,163.83 | v247.65,163.83 v246.38,165.1 246.38,166.37 252.73,166.37 | v247.65,167.64 v247.65,163.83 | 306.07,147.32 321.31,147.32 | v274.64,166.37 v271.78,163.51 | v274.64,163.51 v271.78,163.51 | v271.78,163.51 271.78,163.83
  Bottom 0.813: C45.+ C46.2 | 80.01,164.47 74.93,164.78 v74.93,163.83
  Bottom 1.016: C43.+ C44.2
  Bottom 1.676: v74.93,163.83 74.93,164.47 80.01,164.47 82.55,162.56 82.55,156.21 80.01,153.67 80.01,149.86 76.2,147.32 74.93,146.05 74.93,143.51
  Bottom 1.778: 260.35,144.78 267.97,147.32 269.24,147.32 | IC10.3 269.24,147.32 | 269.24,147.32 283.21,147.32 285.75,146.05 285.75,140.97 | 285.75,140.97 R75.1 | R72.2 287.02,140.97 285.75,140.97 | R73.2 303.53,144.78 306.07,147.32 309.88,147.32 | IC11.3 309.88,147.32 | 309.88,147.32 321.31,147.32 323.85,144.78 328.93,144.78 | 328.93,144.78 R74.2 | 31.75,146.05 15.24,146.05 | 12.7,144.78 8.89,144.78 | 10.16,163.83 v19.05,163.83 | R71.2 260.35,144.78 | 260.35,144.78 259.08,146.05 259.08,154.94 257.81,156.21 257.81,166.37 | 328.93,144.78 328.93,147.32 332.11,158.43 327.66,163.83 314.96,163.83 v314.96,165.1
  Bottom 1.93: R5.1 33.02,140.97 | 33.02,140.97 34.29,139.7 R2.2 | 33.02,140.97 33.02,144.78 31.75,146.05 17.78,146.05 | 17.78,146.05 15.24,146.05 12.7,144.78 11.43,144.78 | IC1.3 17.78,146.05 | R3.2 52.07,143.51 55.88,146.05 58.42,146.05 | 58.42,146.05 72.39,146.05 74.93,143.51 77.47,143.51 R4.2 | IC2.3 58.42,146.05 | R31.1 116.84,140.97 | 116.84,140.97 119.38,140.97 R28.2 | 101.6,147.32 115.57,147.32 116.84,146.05 116.84,140.97 | R27.2 97.79,142.24 97.79,146.05 99.06,147.32 | 99.06,147.32 101.6,147.32 | R30.2 162.56,147.32 | 162.56,147.32 142.24,147.32 | IC5.3 142.24,147.32 | 142.24,147.32 138.43,147.32 135.89,144.78 R29.2 | 184.15,147.32 IC7.3 | R48.2 204.47,144.78 200.66,147.32 184.15,147.32 | 184.15,147.32 179.07,147.32 177.8,146.05 R32.2 177.8,149.86 173.99,156.21 173.99,163.83 v172.72,163.83 166.37,163.83 165.1,161.29 165.1,154.94 162.56,147.32 | 246.38,144.78 242.57,147.32 226.06,147.32 | IC8.3 226.06,147.32 | 226.06,147.32 223.52,147.32 220.98,144.78 220.98,140.97 R49.2 | R1.2 11.43,144.78 | 11.43,144.78 8.89,144.78 8.89,160.02 10.16,163.83 C42.2 | v93.98,165.1 95.49,164.67 | 95.49,164.67 96.2,164.47 102.87,164.47 | IC4.3 101.6,147.32 | 99.06,147.32 97.79,147.32 92.71,152.4 92.71,157.48 95.25,162.56 95.49,164.67 | 246.38,144.78 246.38,146.05 248.92,154.94 248.92,160.02 247.65,162.56 v247.65,163.83 | R50.2 246.38,144.78 | v189.23,165.1 190.5,163.83
  Bottom 2.184: v19.05,163.83 v19.05,167.64 | v175.26,163.83 v172.72,163.83 v187.96,163.83 v189.23,165.1 | v274.64,166.37 257.81,166.37 252.73,166.37 | 252.73,166.37 247.65,166.37 | C48.2 252.73,166.37
  pour Top: 96.52,167.64 96.52,165.1 95.25,163.83 92.71,163.83 91.44,165.1 91.44,167.64
  pour Bottom: 102.87,165.1 103.19,165.42 105.73,165.42 106.68,164.47 106.68,162.56 106.36,162.24 102.87,162.24
  pour Bottom: 102.87,165.1 103.19,165.42 105.73,165.42 106.68,164.47 106.68,162.56 106.36,162.24 102.87,162.24
  pour Top: 102.87,165.1 103.19,165.42 105.73,165.42 106.68,164.47 106.68,162.56 106.36,162.24 102.87,162.24
  pour Top: 170.18,164.15 175.26,169.23 175.58,169.23 175.58,163.51 170.18,163.51
  pour Top: 172.72,166.37 172.72,173.99 175.26,173.99 175.26,166.37
  pour Top (no thermals): 143.51,166.37 140.97,163.83 146.05,163.83
  pour Top: 187.01,162.56 191.45,162.56 191.77,162.88 191.77,166.05 191.45,166.37 187.01,166.37 186.69,166.05 186.69,162.88
  pour Bottom: 187.01,162.56 191.45,162.56 191.77,162.88 191.77,166.05 191.45,166.37 187.01,166.37 186.69,166.05 186.69,162.88
  pour Top: 248.92,169.23 248.92,163.51 247.97,162.88 245.11,162.88 244.47,163.51 244.47,166.05 246.38,169.23
  pour Bottom: 248.92,169.23 248.92,163.51 247.97,162.88 245.11,162.88 244.47,163.51 244.47,166.05 246.38,169.23
  pour Bottom: 276.86,166.37 276.86,162.56 276.54,162.24 270.83,162.24 270.83,165.1 273.69,167 276.86,167
  pour Top: 276.86,166.37 276.86,162.56 276.54,162.24 270.83,162.24 270.83,165.1 273.69,167 276.86,167
  pour Top (no thermals): 315.91,166.37 315.91,163.51 310.83,163.51 314.32,170.18 314.96,170.81 315.6,170.18 315.91,169.86
  pour Bottom (no thermals): 315.91,166.37 315.91,163.51 310.83,163.51 314.32,170.18 314.96,170.81 315.6,170.18 315.91,169.86
-12V
  Top 1.016: C68.2 63.5,76.2 65.09,77.79 65.09,82.87 74.93,92.71 74.93,109.22 67.31,116.84 67.31,120.65 66.04,121.92 R26.1
  Bottom 0.813: R26.1 66.04,119.38 129.54,119.38 | 129.54,119.38 R52.1 | 129.54,119.38 130.81,118.11 173.99,118.11 173.99,119.38
  Bottom 1.016: R70.1 173.99,119.38 227.33,119.38 R92.1 | C68.2 58.42,76.2 58.42,71.12 53.34,76.2 DC1.4
GND  (via drill 0.6)
  Top 0.406: 86.36,138.43 D8.A | U$1.2 R23.2 | C15.1 C12.1 v147.32,130.81 | IC9.3 153.67,113.03 156.21,113.03 IC9.5 158.75,113.03 | C27.2 165.1,113.03 158.75,113.03 | U3.5 157.48,101.6 158.75,102.87 158.75,113.03 | 203.2,137.16 208.28,137.16 D20.A | C35.2 226.06,123.83 227.33,125.73 229.87,125.73 231.14,127 231.14,129.54 v232.41,130.81 | OK1.3 279.4,124.46 281.94,124.46 284.48,127 292.1,127 293.37,128.27 D28.A | v214.63,46.99 v214.63,97.79 | IC16.1 114.3,50.8 114.3,30.48 IC16.10 | IC15.23 144.78,17.78 v138.43,17.78 | OK7.5 215.9,24.13 203.2,24.13 | C72.1 95.57,79.06 95.57,82.87 C20.2 | C77.2 DC1.2
  Top 0.61: v200.66,137.16 203.2,137.16 204.47,134.62 220.98,134.62 v222.25,135.89 | C35.2 221.61,120.33 221.61,115.25 C36.2 222.25,102.87 224.79,100.33 U4.1 | v214.63,46.99 C52.2 | IC14.16 184.15,48.26 185.42,49.53 v185.42,88.9 | IC26.3 IC26.4 | IC27.15 63.5,16.51 C66.2
  Top 0.813: C8.2 C9.2 55.88,111.76 58.42,109.22 63.5,109.22 C7.1 | C18.2 120.65,120.65 120.65,115.57 C19.2 | C26.2 165.1,120.65 165.1,115.57 C27.2 | v274.32,130.81 C31.1 276.86,140.97 R76.1 | v251.46,130.81 D24.A | D28.A 295.91,138.43 | D31.A 295.91,138.43 | 295.91,138.43 295.91,160.02 | C41.- 16.13,168.53 C42.1 | C52.2 v214.63,97.79 | C28.2 143.51,93.98 v144.78,92.71 | v153.35,92.71 153.35,79.38 IC13.16 IC20.1 149.86,66.04 149.86,43.18 IC20.10 v151.13,29.21 | IC21.10 233.68,58.42 C55.2 233.68,92.71 234.95,93.98 U4.5 | R102.2 R103.2 | U2.5 113.03,95.25 107.95,90.17 v107.95,83.82 | IC16.10 C38.2 v113.03,21.91 | v121.92,21.91 v121.92,17.78 SV1.2 | 204.47,31.75 204.47,30.48 203.2,29.21 OK9.5 203.2,24.13 190.5,24.13 | IC18.10 204.47,31.75 | 204.47,31.75 C56.2 | 185.42,24.13 190.5,24.13 | OK6.9 190.5,24.13 | OK6.11 185.42,24.13 | 185.42,24.13 184.15,22.86 180.34,22.86 | OK6.13 180.34,22.86 | OK6.15 175.26,24.13 | 175.26,24.13 171.77,24.13 171.13,24.77 171.13,27.62 JP1.1 | IC15.2 IC15.1 | v175.26,21.27 175.26,22.86 | 175.26,24.13 175.26,22.86 | 175.26,22.86 180.34,22.86 | IC23.25 81.28,50.8 IC23.36 | IC23.2 IC23.68 | C60.1 103.19,8.89 104.14,9.84 v104.14,26.04 | DC1.5 51.44,78.74 52.07,78.11 52.07,71.76 51.44,71.12 DC1.2 | C69.1 LSP1.MP C70.1 82.55,83.82 v77.47,83.82 | v48.26,64.77 v48.26,59.69 | OK3.7 90.17,109.22 94.61,104.78 94.61,84.77 93.66,83.82 C59.-
  Top 1.016: 44.45,160.02 44.45,138.43 D4.A IC3.12 41.91,120.65 | 86.36,160.02 86.36,138.43 | 41.91,120.65 IC3.3 41.91,113.03 45.72,113.03 | IC3.5 45.72,113.03 | 41.91,120.65 45.72,120.65 IC3.10 | 45.72,113.03 45.72,100.33 U1.1 46.99,95.25 U$1.2 | 128.27,160.02 128.27,138.43 D12.A | D16.A 170.18,138.43 | 170.18,138.43 170.18,160.02 | IC6.3 107.95,115.57 | 107.95,115.57 107.95,120.65 | 107.95,120.65 IC6.12 v107.95,132.08 R33.1 | 107.95,115.57 113.03,115.57 IC6.5 | 107.95,120.65 111.76,120.65 IC6.10 | 170.18,138.43 D19.A | D24.A 254,138.43 | 254,138.43 254,160.02 | R56.1 236.22,137.16 233.68,134.62 C21.1 C24.1 | IC9.12 152.4,119.38 | 152.4,119.38 IC9.3 | 152.4,119.38 156.21,119.38 157.48,120.65 IC9.10 | D27.A 254,138.43 | D32.A 336.55,140.97 336.55,156.21 332.74,160.02 320.04,160.02 | IC12.12 209.55,120.65 | 209.55,120.65 209.55,115.57 | 209.55,115.57 IC12.3 | IC12.5 213.36,115.57 209.55,115.57 | IC12.10 213.36,120.65 209.55,120.65 | C48.1 257.81,172.66 C47.- | C49.- 320.04,172.66 C50.1 | C58.- 253.75,54.86 255.27,53.34 260.35,53.34 SV2.2 R116.1 | SV6.2 65.41,62.87 v66.04,63.5 IC23.14 | C67.2 60.96,93.98 U1.5 | C73.2 91.76,37.78 | v91.76,34.29 91.76,37.78 | 91.76,37.78 93.98,35.56 93.98,32.7 92.71,31.43 v92.71,26.04 | IC23.27 72.39,45.72 71.44,44.77 71.44,35.88 v70.48,35.24 | C75.2 C76.-
  Top 1.27: C87.2 D54.A 13.97,34.29
  Top 1.422: D11.A D8.A | D23.A 212.09,138.43 212.09,160.02
  Top 1.778: C42.1 15.24,160.02 | C48.1 257.81,160.02
  Top 1.93: C44.1 80.01,160.02 | C46.1 100.33,160.02
  Top 2.184: D3.A 3.81,140.97 3.81,160.02 15.24,160.02 24.13,160.02 | 24.13,160.02 IC1.8 | 24.13,160.02 44.45,160.02 64.77,160.02 | IC2.8 64.77,160.02 | 64.77,160.02 80.01,160.02 86.36,160.02 100.33,160.02 107.95,160.02 | IC4.8 107.95,160.02 | 107.95,160.02 128.27,160.02 148.59,160.02 | 148.59,160.02 IC5.8 | 148.59,160.02 170.18,160.02 180.34,160.02 | 180.34,160.02 190.5,160.02 | IC7.8 190.5,160.02 | 190.5,160.02 212.09,160.02 232.41,160.02 | 232.41,160.02 IC8.8 | 232.41,160.02 254,160.02 257.81,160.02 275.59,160.02 | IC10.8 275.59,160.02 | IC11.8 316.23,160.02 | 316.23,160.02 295.91,160.02 275.59,160.02 | 316.23,160.02 320.04,160.02 C50.1 | X5.1 180.34,160.02 | B3.- 8.8,52.16 11.43,49.53 11.43,36.83 13.97,34.29 11.43,31.75 5.08,31.75 3.81,30.48 D52.A
  Bottom 0.406: IC3.3 43.18,113.03 54.61,113.03 C9.2 | C10.2 43.18,99.06 46.99,99.06 | R33.1 113.03,138.43 118.11,138.43 119.38,137.16 124.46,137.16 D12.A | v147.32,130.81 111.76,130.81 109.22,132.08 v107.95,132.08 | C19.2 120.65,115.57 114.3,115.57 IC6.5 | U2.5 111.76,98.74 104.14,98.74 U2.1 | IC12.5 215.9,115.57 220.98,115.57 C36.2 | v232.41,130.81 v251.46,130.81 | OK3.4 82.55,124.46 82.55,138.43 | v214.63,97.79 IC17.10 | v138.43,17.78 v121.92,17.78 | IC25.5 IC25.6 IC25.7 IC25.5 | IC25.5 83.5,39.37 83.5,33.02 83.48,32.28 | QF1.2 77.44,81.25 LSP1.MP QF1.2
  Bottom 0.61: C3.1 24.13,137.16 26.03,137.16 R7.1 31.75,137.16 38.1,137.16 39.37,135.89 54.61,135.89 55.88,137.16 63.5,137.16 | 63.5,137.16 68.58,137.16 68.58,138.43 | 68.58,138.43 R9.1 | 68.58,138.43 82.55,138.43 D8.A | C5.1 63.5,137.16 | 63.5,137.16 C2.1 | R54.1 v200.66,137.16 | C21.1 228.6,135.89 v222.25,135.89 | U4.1 224.79,99.06 | OK2.5 72.39,115.57 77.47,115.57 | OK2.7 77.47,115.57 | 77.47,115.57 85.09,115.57 | OK3.5 85.09,115.57 | 85.09,115.57 90.17,115.57 OK3.7 | IC19.14 203.2,46.99 v214.63,46.99
  Bottom 0.813: C13.1 109.22,135.89 R33.1 | R54.1 191.77,140.97 189.23,138.43 C22.1 | 147.32,99.06 144.78,99.06 C28.2 | U3.1 147.32,99.06 | v251.46,130.81 v274.32,130.81 276.86,129.54 307.34,129.54 C30.1 314.96,137.16 | C33.1 314.96,137.16 | R78.1 320.04,138.43 318.77,137.16 314.96,137.16 | 234.95,99.06 224.79,99.06 223.52,99.06 C37.2 v214.63,97.79 C39.2 IC17.10 203.2,99.06 157.48,99.06 | 234.95,99.06 U4.5 | C45.- 97.79,168.91 C46.1 | OK5.7 265.43,115.57 261.62,115.57 | OK5.5 261.62,115.57 | 261.62,115.57 252.73,115.57 | 252.73,115.57 OK4.7 252.73,100.33 236.22,100.33 234.95,99.06 | 252.73,115.57 247.65,115.57 OK4.5 | U3.5 157.48,99.06 | 157.48,99.06 147.32,99.06 | v144.78,92.71 v153.35,92.71 | C52.2 213.36,88.9 C57.2 v185.42,88.9 176.53,88.9 175.26,90.17 168.91,90.17 167.64,88.9 R102.2 | R103.2 156.53,81.28 C54.2 156.21,81.6 110.17,81.6 v107.95,83.82 v107.31,83.82 C20.2 C59.- 86.36,83.82 | v113.03,21.91 v121.92,21.91 | JP1.1 164.46,29.21 163.19,30.48 151.13,30.48 v151.13,29.21 | C51.2 179.39,35.56 203.2,35.56 IC18.10 | IC15.2 163.83,16.51 166.37,19.05 169.23,19.05 171.45,21.27 v175.26,21.27 | IC23.2 IC23.4 IC23.6 | IC23.6 IC23.8 IC23.11 IC23.10 IC23.12 IC23.14 69.85,63.5 68.9,62.55 68.9,51.75 69.85,50.8 IC23.24 | IC23.5 IC23.7 IC23.9 | IC23.3 IC23.5 | IC23.5 IC23.6 | IC23.25 IC23.24 | IC23.24 IC23.26 71.12,46.99 72.39,45.72 IC23.27 | C60.1 SV5.1 | C71.2 86.36,80.01 86.36,83.82 | 86.36,83.82 86.36,84.46 85.41,85.41 78.74,85.41 77.47,84.14 v77.47,83.82 | IC26.3 61.59,31.75 53.34,31.75 50.8,29.21 C64.+ | v48.26,64.77 49.21,65.72 49.21,70.17 50.16,71.12 DC1.2 | D52.A 7.62,24.13 R126.2 | IC27.15 60.96,12.7 60.33,12.07 50.39,12.07
  Bottom 0.813: 42.55,13.02 43.5,12.07 50.39,12.07 | C88.- 42.55,13.02 | 42.55,13.02 40.96,11.43 31.75,11.43 31.75,12.7 | 50.39,12.07 X14.5 | C86.- 34.29,29.21 | 73.34,26.04 71.12,27.94 71.12,30.48 66.36,33.66 IC26.4
  Bottom 1.016: D4.A D7.A | U1.1 46.99,99.06 55.88,99.06 U1.5 | C15.1 149.86,140.97 R35.1 | D20.A D23.A | D33.A 158.75,171.45 C53.- | C43.- 80.01,171.45 C44.1 | IC15.23 156.21,16.51 IC15.1 | 248.92,56.52 C58.- | IC22.9 248.92,56.52 | 248.92,56.52 234.95,56.52 233.04,58.42 IC21.10 | DC1.5 C68.1 62.23,78.74 62.86,79.38 62.86,83.19 | 62.86,83.19 62.23,83.82 | 62.23,83.82 66.04,83.82 68.58,81.28 | 62.86,83.19 62.86,83.5 62.23,83.82 | 62.23,83.82 C67.2 | C74.2 83.19,32.07 | 83.19,32.07 83.48,32.28 86.36,34.29 v91.76,34.29 | v70.48,35.24 70.48,34.29 72.71,32.07 83.19,32.07
  Bottom 1.27: C53.- C40.1 179.07,171.45 180.34,172.72 X5.1 | IC26.4 71.12,30.48 71.12,28.26 73.34,26.04 v92.71,26.04 v104.14,26.04 C38.2 | SV7.2 35.56,30.48
  Bottom 1.422: D12.A D15.A
  Bottom 1.778: C75.2 44.45,53.34 42.86,51.75 42.86,36.83
  Bottom 1.93: v77.47,83.82 71.12,83.82 68.58,81.28 68.58,66.04 v66.04,63.5 D45.A 52.07,63.5 v48.26,59.69 45.4,56.83 C75.2
  Bottom 2.184: 34.29,29.21 35.56,30.48 41.59,36.51 63.82,36.51 66.04,34.29 IC26.4
  other vias: 121.92,114.3 231.14,134.62 143.51,97.79 77.47,81.28 60.96,83.82 90.17,114.3
  pour Top: 44.45,157.48 41.91,160.02 46.99,160.02
  pour Top: 86.36,157.48 83.82,160.02 88.9,160.02
  pour Top: 128.27,157.48 125.73,160.02 130.81,160.02
  pour Top: 170.18,157.48 167.64,160.02 172.72,160.02
  pour Top: 212.09,157.48 209.55,160.02 214.63,160.02
  pour Top: 251.46,160.02 254,157.48 256.54,160.02
  pour Top: 295.91,157.48 293.37,160.02 297.18,160.02 298.45,160.02
  pour Top: 12.7,160.02 15.24,162.56 17.78,160.02
  pour Top: 180.34,162.56 177.8,160.02 182.88,160.02
  pour Top (no thermals): 149.54,64.14 149.54,69.85 150.49,70.8 150.49,76.84 153.35,79.69 153.35,82.55 155.26,82.55 155.89,81.28 156.53,80.96 156.53,79.69 153.03,75.57 153.03,66.04 151.76,64.14
  pour Top: 106.68,83.82 106.68,84.14 107,84.46 108.9,84.46 109.22,84.14 109.22,83.5 108.9,83.19 107,83.19 106.68,83.5
  pour Bottom: 106.68,83.82 106.68,84.14 107,84.46 108.9,84.46 109.22,84.14 109.22,83.5 108.9,83.19 107,83.19 106.68,83.5
  pour Bottom (no thermals): 15.87,35.24 15.87,33.66 28.26,21.27 28.26,13.65 30.8,11.11 34.61,11.11 34.61,29.53 26.67,29.53 20.95,35.24
GND1  (via drill 0.6)
  Top 0.406: C83.2 D51.A | OK3.2 90.17,123.19 88.9,124.46 78.74,124.46 77.47,123.19
  Top 0.813: OK2.2 77.47,123.19 73.66,123.19 OK2.4 | v33.02,129.54 31.75,128.27 31.75,124.46 26.67,119.38 26.67,87.63 25.4,86.36 25.4,81.28 D51.A
  Top 1.676: IC29.GND 24.13,55.88 25.4,57.15 25.4,69.85 C82.-
  Bottom 0.406: 5.08,68.58 C85.2 | D49.A C84.-
  Bottom 0.813: OK2.4 64.77,129.54 v33.02,129.54
  Bottom 1.676: B2.- 40.64,77.47 31.75,77.47 | C82.- 31.75,77.47 | 31.75,77.47 D51.A 21.59,76.2 13.97,68.58 X15.8 5.08,68.58 | IC29.GND 24.13,55.88 28.19,59.94 C84.-
N$1  (via drill 0.6)
  Top 0.406: IC1.13 R5.2 v36.83,143.51 | v71.12,142.24 IC2.13
  Bottom 0.406: v36.83,143.51 39.37,140.97 46.99,140.97 49.53,138.43 53.34,138.43 54.61,139.7 54.61,140.97 55.88,142.24 v71.12,142.24
N$2
  Bottom 0.406: X1.2 39.37,171.45
  Bottom 1.422: IC1.15 34.29,151.13 | 39.37,171.45 39.37,168.91 34.29,160.02 34.29,151.13 | 34.29,151.13 38.1,147.32 D2.A D4.C
N$3
  Top 1.422: D5.A 48.26,149.86 IC2.1
  Bottom 1.422: D7.C D5.A | X1.3 41.91,161.29 43.18,160.02 53.34,160.02 54.61,158.75 54.61,151.13 IC2.1
N$4
  Top 1.422: D6.A 81.28,149.86 IC2.15
  Bottom 1.422: X1.4 45.72,162.56 54.61,162.56 57.15,160.02 73.66,160.02 74.93,158.75 74.93,151.13 IC2.15 | D6.A D8.C
N$5
  Top 0.406: IC1.5 20.32,148.59 17.78,146.05 R10.2
N$6
  Top 1.422: IC2.14 R4.1 82.55,154.94 D6.C
N$7
  Top 1.422: D1.A 8.89,149.86 IC1.1
  Bottom 1.422: D3.C D1.A | IC1.1 13.97,151.13 13.97,158.75 15.24,160.02 29.21,160.02 X1.1
N$8
  Top 0.406: IC1.11 R7.2 26.67,142.24 26.67,139.7 R8.1
N$9
  Top 1.422: IC1.14 R2.1
  Bottom 1.422: D2.C 40.64,153.67 39.37,154.94 R2.1
N$10
  Top 1.422: R3.1 IC2.2
  Bottom 1.422: D5.C 48.26,154.94 R3.1
N$11
  Top 1.422: IC1.2 R1.1 7.62,154.94 D1.C
N$12  (via drill 0.6)
  Top 0.406: IC1.4 21.59,152.4 v21.59,135.89
  Bottom 0.406: C1.2 R8.2 v21.59,135.89
N$13
  Top 0.406: IC2.4 59.69,148.59 57.15,146.05 57.15,134.62 C2.2
  Bottom 0.406: C1.1 36.83,134.62 C2.2 | IC2.4 60.96,157.48 66.04,157.48 IC2.10
N$14
  Top 0.406: IC2.11 R9.2
N$15  (via drill 0.6)
  Top 0.406: IC1.12 v29.21,134.62 | IC2.12 v69.85,133.35 | IC4.12 113.03,153.67 115.57,151.13 115.57,147.32 118.11,144.78 118.11,138.43 v121.92,134.62 | R6.2 77.47,132.08 80.01,132.08 82.55,134.62 v102.87,134.62 | IC5.12 156.21,151.13 v156.21,135.89 | IC7.12 195.58,144.78 196.85,143.51 196.85,137.16 199.39,134.62 v199.39,130.81 | IC11.12 v321.31,128.27 | IC8.12 v237.49,134.62 | 280.67,144.78 IC10.12 v280.67,134.62 v280.67,128.27 280.67,127 279.4,125.73 278.13,125.73 276.86,124.46 OK1.4
  Bottom 0.406: v29.21,134.62 30.48,134.62 31.75,133.35 v69.85,133.35 71.12,134.62 R6.2 | v102.87,134.62 104.14,133.35 110.49,133.35 113.03,134.62 v121.92,134.62 137.16,134.62 138.43,135.89 v156.21,135.89 165.1,135.89 166.37,134.62 190.5,134.62 193.04,130.81 v199.39,130.81 207.01,130.81 209.55,133.35 228.6,133.35 229.87,132.08 232.41,132.08 233.68,133.35 236.22,133.35 v237.49,134.62 238.76,133.35 260.35,133.35 261.62,134.62 v280.67,134.62 | v280.67,128.27 v321.31,128.27
N$16
  Bottom 0.406: R11.1 R10.1 C3.2
N$17
  Top 0.406: IC1.7 R12.2
  Bottom 0.406: R11.2 R12.2
N$18
  Bottom 0.406: R12.1 C4.1
N$19
  Top 0.406: IC1.9 C4.2
N$20
  Top 0.406: R13.2 58.42,146.05 60.96,148.59 IC2.5
N$21
  Bottom 0.406: C5.2 R13.1 R14.1
N$22
  Top 0.406: IC2.7 R15.2
  Bottom 0.406: R14.2 R15.2
N$23
  Bottom 0.406: R15.1 C6.1
N$24
  Top 0.406: IC2.9 C6.2
N$25  (via drill 0.6)
  Top 0.406: v52.07,111.76 IC3.7 53.34,115.57 53.34,125.73 v54.61,127 | v24.13,151.13 v24.13,129.54
  Bottom 0.406: v52.07,111.76 R16.2 | IC1.6 v24.13,151.13 | v24.13,129.54 30.48,129.54 31.75,128.27 49.53,128.27 v49.53,127 v54.61,127
N$26
  Top 0.406: IC3.6 R16.1 | R18.2 R17.2
  Bottom 0.406: R16.1 R17.2
N$27  (via drill 0.6)
  Top 0.406: IC3.1 R17.1 38.1,111.76 40.64,109.22 v40.64,106.68 | U1.3 48.26,101.6 v48.26,106.68
  Bottom 0.406: v48.26,106.68 v40.64,106.68
N$28  (via drill 0.6)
